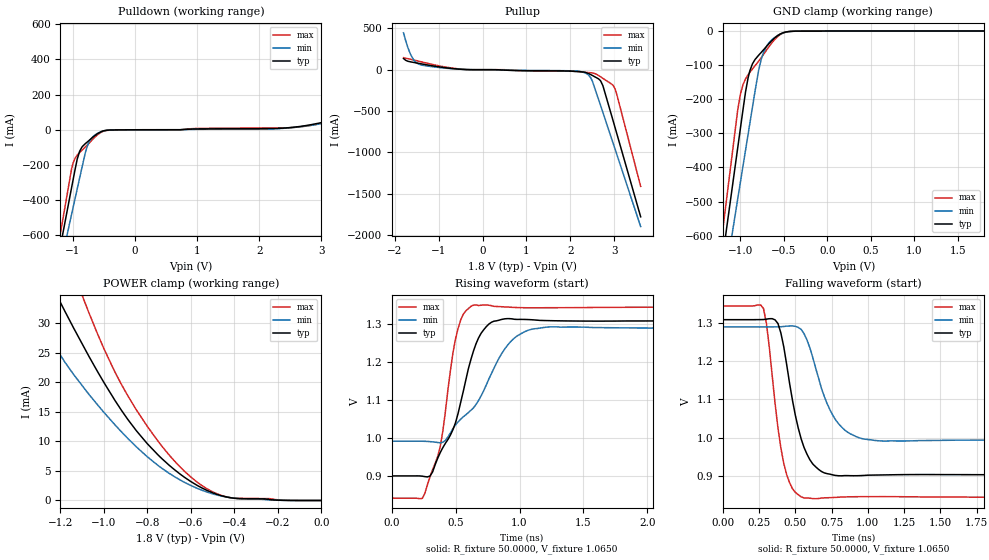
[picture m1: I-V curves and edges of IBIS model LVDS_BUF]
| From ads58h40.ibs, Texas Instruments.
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|   Model LVDS_BUF
[Model]  LVDS_BUF
Model_type 3-state
Polarity   Non-Inverting
Enable   Active-Low
Vmeas =  1.2V
C_comp   2.5000pF   2.2500pF   2.7500pF
[Temperature Range]   25.0000   0.1250k   -40.0000
[Voltage Range]   1.8000V   1.7000V   2.0000V
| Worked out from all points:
|   slope of the pulldown table from 0 to 0.27 V, typ, clamps not added: 2.06 kohm
|   slope of the pullup table from 0 to 0.27 V, typ, clamps not added: 19 kohm
|   GND clamp passes 1 mA (typ) near -0.42 V on its own axis
|   POWER clamp passes 1 mA (typ) near -0.48 V on its own axis
|   rising waveform, R_fixture 50.0000, V_fixture 1.0650: 20-80 % time 225ps typ, 331ps min, 140ps max; typ from 0.901 V to 1.31 V
|   falling waveform, R_fixture 50.0000, V_fixture 1.0650: 20-80 % time 128ps typ, 165ps min, 96.8ps max; typ from 1.31 V to 0.901 V
[Pulldown]
|Voltage   I(typ)   I(min)   I(max)
-1.8V     -1.771A    -1.732A    -1.811A
-1.02V    -328mA     -479.8mA   -220.8mA
-890mV    -121.6mA   -273.1mA   -129.2mA
-770mV    -70.41mA   -95.96mA   -88.16mA
-690mV    -46.15mA   -44.05mA   -57.94mA
-520mV    -7.954mA   -8.025mA   -10.02mA
2.32V     7.654mA    6.289mA    10.2mA
3.16V     51.94mA    60.18mA    51.12mA
3.33V     63.36mA    166.6mA    68.7mA
3.44V     74.63mA    326.2mA    80.01mA
3.57V     107.6mA    595.5mA    90.92mA
3.6V      123.2mA    666.3mA    93.3mA
[Pullup]
|Voltage   I(typ)   I(min)   I(max)
-1.8V     135.1mA    446.1mA    145.3mA
-1.64V    94.92mA    185mA      126.6mA
-1.54V    85.13mA    101.4mA    114.1mA
-1.42V    73.1mA     61.24mA    98.52mA
-400mV    2.455mA    2.983mA    2.858mA
2.23V     -24.89mA   -21.83mA   -24.69mA
2.46V     -57.88mA   -94.82mA   -36.63mA
2.64V     -110.9mA   -357.9mA   -68.98mA
2.74V     -193.1mA   -516.9mA   -104.7mA
2.94V     -557.8mA   -836.4mA   -173.9mA
3.02V     -705.4mA   -964.6mA   -236.4mA
3.6V      -1.778A    -1.897A    -1.41A
[GND_clamp]
|Voltage   I(typ)   I(min)   I(max)
-1.8V     -1.766A    -1.727A    -1.805A
-1.03V    -342.9mA   -492.8mA   -232mA
-1V       -287.7mA   -445mA     -186.7mA
-970mV    -232.5mA   -397.3mA   -157.9mA
-910mV    -136.7mA   -302.2mA   -128.1mA
-860mV    -96.09mA   -223.1mA   -111.1mA
-790mV    -71.3mA    -116.3mA   -88.73mA
-760mV    -62.89mA   -83.49mA   -78.39mA
-690mV    -42.57mA   -41.25mA   -52.97mA
-570mV    -13.32mA   -12.85mA   -16.19mA
-360mV    -391.4uA   -482uA     -482.9uA
1.8V      55.44nA    3.177uA    33.91pA
[POWER_clamp]
|Voltage   I(typ)   I(min)   I(max)
-1.8V     117.3mA    440.3mA    111.9mA
-1.33V    43.1mA     34.45mA    57.88mA
-1.22V    34.98mA    25.77mA    46.53mA
-1.18V    32.09mA    23.46mA    42.5mA
-1.14V    29.27mA    21.38mA    38.55mA
-1.07V    24.49mA    18.03mA    31.89mA
-950mV    17mA       12.85mA    21.82mA
-850mV    11.79mA    9.06mA     15.31mA
-700mV    5.978mA    4.609mA    7.714mA
-570mV    2.537mA    2.045mA    3.081mA
-410mV    429.4uA    431.2uA    428.5uA
0V        55.44nA    189.1nA    22.56nA
[Ramp]
| variable   typ   min   max
dV/dt_r  0.365/94.7491p   0.269/0.1191n   0.457/86.5313p
dV/dt_f  0.151/0.1295n   0.081/0.1224n   0.2483/0.1671n
R_load = 50.0000
[Rising Waveform]
R_fixture= 50.0000
V_fixture= 1.0650
V_fixture_min= 1.1050
V_fixture_max= 1.0450
|time   V(typ)   V(min)   V(max)
0s        901.5mV    992.6mV    843.1mV
260ps     899.6mV    992.3mV    856mV
380ps     962.8mV    988.5mV    978.6mV
480ps     1.024V     1.026V     1.227V
520ps     1.066V     1.044V     1.29V
640ps     1.23V      1.08V      1.35V
760ps     1.3V       1.156V     1.35V
940ps     1.314V     1.258V     1.344V
1.24ns    1.309V     1.293V     1.343V
20ns      1.309V     1.29V      1.345V
[Falling Waveform]
R_fixture= 50.0000
V_fixture= 1.0650
V_fixture_min= 1.1050
V_fixture_max= 1.0450
|time   V(typ)   V(min)   V(max)
0s        1.309V     1.29V      1.345V
280ps     1.309V     1.29V      1.338V
380ps     1.299V     1.29V      1.025V
420ps     1.238V     1.291V     932.5mV
480ps     1.098V     1.293V     866mV
540ps     996.8mV    1.284V     844.9mV
620ps     931mV      1.21V      840.3mV
800ps     900.1mV    1.036V     843.9mV
1.1ns     902.2mV    991.1mV    845.4mV
20ns      901.4mV    992.6mV    843mV
